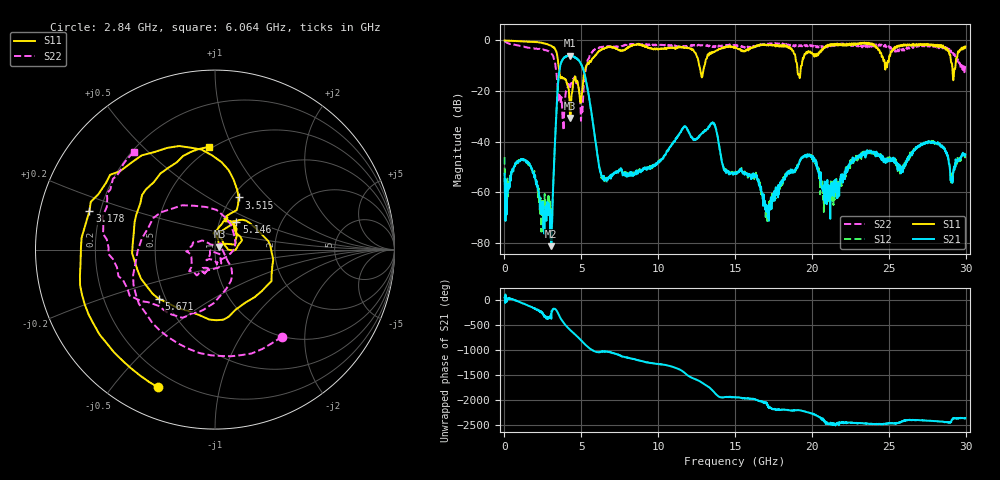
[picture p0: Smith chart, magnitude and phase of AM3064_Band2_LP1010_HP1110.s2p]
# Hz S DB R 50.0
!freq dBS11 angS11 dBS21 angS21 dBS12 angS12 dBS22 angS22
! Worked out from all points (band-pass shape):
!   1600 points, 10 MHz to 29.98 GHz, reference 50 ohm
!   highest |S21| = -5.98 dB at 4.265 GHz (marker M1); lowest = -81.2 dB at 3.046 GHz (marker M2)
!   |S21| within 3 dB of the highest: 3.678 GHz to 4.95 GHz (1.272 GHz wide, 29.5 % of centre)
!   lowest |S11| = -30.6 dB at 4.284 GHz (marker M3), VSWR 1.06, Z = 52.5 + j1.7 ohm
!   |S11| at or under -10 dB: 3.516 GHz to 5.333 GHz (1.817 GHz wide, 41.1 % of centre); 12.67 GHz to 13.01 GHz (338.5 MHz wide, 2.64 % of centre); 19.04 GHz to 19.33 GHz (288.1 MHz wide, 1.5 % of centre)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
!   |S22| runs from -35.5 to -0.3 dB; largest |S21 - S12| = 0.016
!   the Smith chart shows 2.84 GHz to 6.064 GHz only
!   S11 on the Smith chart (normalised r, x): 2.84 GHz: 0.13, -0.66; 3.178 GHz: 0.16, +0.15; 3.515 GHz: 1.07, +0.69; 5.146 GHz: 1.20, +0.39; 5.671 GHz: 0.46, -0.30; 6.064 GHz: 0.48, +0.82
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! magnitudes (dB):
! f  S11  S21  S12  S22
! 10 MHz  0.0  -52.6  -46.1  -0.3
! 1.435 GHz  -0.4  -48.3  -47.8  -2.7
! 2.84 GHz  -1.6  -68.8  -65.4  -4.3
! 3.046 GHz  -2.1  -81.2  -70.3  -5.1
! 3.178 GHz  -2.7  -55.7  -56.1  -6.4
! 3.515 GHz  -9.9  -14.8  -14.9  -22.6
! 3.796 GHz  -15.0  -7.4  -7.3  -31.6
! 4.265 GHz  -30.2  -6.0  -6.1  -19.0
! 4.284 GHz  -30.6  -6.1  -5.9  -18.2
! 5.015 GHz  -22.0  -9.8  -9.6  -27.2
! 5.146 GHz  -14.1  -11.9  -12.0  -18.4
! 5.671 GHz  -7.6  -29.2  -29.0  -5.1
! 6.064 GHz  -4.8  -45.5  -45.9  -3.0
! 6.645 GHz  -2.7  -55.3  -56.2  -2.6
! 10 GHz  -3.4  -47.6  -48.2  -1.8
! 13.54 GHz  -4.9  -32.7  -32.4  -2.6
! 15 GHz  -2.6  -52.6  -52.6  -1.8
! 17.09 GHz  -1.8  -65.1  -71.9  -1.6
! 19.99 GHz  -4.8  -45.7  -45.6  -1.9
! 21.04 GHz  -1.9  -57.5  -63.5  -2.1
! 25 GHz  -7.9  -47.2  -47.0  -2.3
! 29.98 GHz  -2.4  -45.1  -45.8  -10.1
